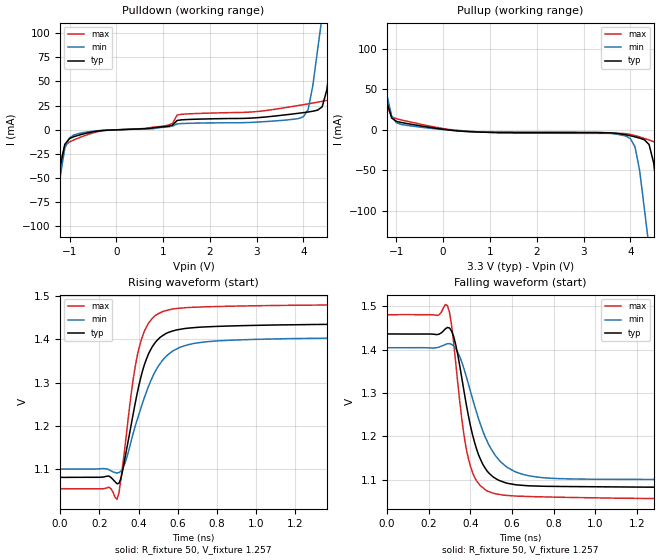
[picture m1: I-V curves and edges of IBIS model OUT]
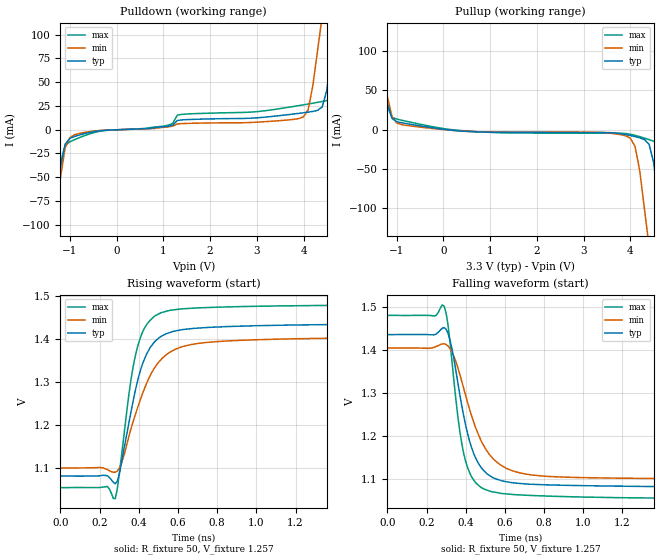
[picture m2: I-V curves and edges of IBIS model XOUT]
[IBIS Ver]   3.2
[Comment Char]   |_char
[File name]   vg3225vfn_lvds.ibs
[File Rev]   1.0
[Date]   2019/07/25 5:37:50
[Source]
[Notes]
[Disclaimer]
Seiko Epson Corporation makes no warranty with respect to the information
contained herein.
[Copyright]
Copyright(C) 2016, Seiko Epson Corporation. All rights reserved.
[Component]   vg3225vfn
Si_location Pin
Timing_location Pin
[Manufacturer]   Seiko Epson Corporation
[Package]
R_pkg   0.048   NA   NA
L_pkg   0.48n   NA   NA
C_pkg   0.21p   NA   NA
[Pin] signal_name   model_name   R_pin   L_pin   C_pin
1   VC   NC
2   OE   NC
3   GND   GND
4   OUT   OUT   0.048   0.48n   0.21p
5   XOUT   XOUT   0.048   0.48n   0.21p
6   VCC   POWER
[Diff Pin] inv_pin vdiff   tdelay_typ
4   5   0   0
| Models and submodels in the file (2): OUT (Output), XOUT (Output)
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[Model]   OUT
Model_type Output
Enable Active-High
Polarity Non-Inverting
Vref=1.250
Vmeas=1.250
Rref=50
Cref=0
C_comp   2.5p   2.5p   2.5p
[Temperature Range] 25   105   -40
[Voltage Range]   3.3   3.0   3.6
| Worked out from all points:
|   slope of the pulldown table from 0 to 0.495 V, typ, clamps not added: 525 ohm
|   slope of the pullup table from 0 to 0.495 V, typ, clamps not added: 178 ohm
|   falling waveform, R_fixture 50, V_fixture 1.257: 20-80 % time 95.8ps typ, 136ps min, 71.1ps max; typ from 1.44 V to 1.08 V
|   rising waveform, R_fixture 50, V_fixture 1.257: 20-80 % time 108ps typ, 149ps min, 84.3ps max; typ from 1.08 V to 1.44 V
[Pullup]
-3.3V     902.7mA    802.4mA    1.011A
-1.5V     156.5mA    150.6mA    165.7mA
-1.4V     115.1mA    114.4mA    118.8mA
-1.2V     33.42mA    42.1mA     29.33mA
-1V       10.35mA    8.744mA    13.55mA
3.9V      -6.214mA   -7.781mA   -4.855mA
4.1V      -8.8mA     -21.11mA   -7.16mA
4.3V      -12.42mA   -97.71mA   -10.64mA
4.5V      -41.27mA   -192.6mA   -14.74mA
4.7V      -144.8mA   -287.5mA   -20.73mA
5V        -306.1mA   -429.9mA   -148.7mA
6.6V      -1.166A    -1.189A    -1.111A
[Pulldown]
-3.3V     -1.17A     -1.051A    -1.295A
-1.4V     -142.7mA   -143.7mA   -146.1mA
-1.3V     -88.9mA    -96.14mA   -85.92mA
-1.2V     -38.72mA   -49.22mA   -34.15mA
-1.1V     -15.04mA   -18.91mA   -16.41mA
-900mV    -7.065mA   -5.272mA   -10.42mA
3.9V      17.07mA    11.65mA    25.14mA
4.1V      18.37mA    21.03mA    26.78mA
4.4V      23.74mA    118.1mA    29.41mA
4.7V      122.4mA    226.4mA    33.54mA
5V        246.7mA    334.8mA    131.6mA
6.6V      911.6mA    915mA      886.2mA
[Falling Waveform]
R_fixture=50
V_fixture=1.257
V_fixture_min=1.251
V_fixture_max=1.265
0s        1.436V     1.405V     1.481V
290ps     1.452V     1.414V     1.502V
330ps     1.411V     1.402V     1.368V
360ps     1.331V     1.37V      1.236V
390ps     1.249V     1.322V     1.149V
430ps     1.17V      1.255V     1.097V
480ps     1.12V      1.189V     1.074V
580ps     1.091V     1.127V     1.063V
740ps     1.085V     1.105V     1.06V
2ns       1.081V     1.1V       1.054V
[Rising Waveform]
R_fixture=50
V_fixture=1.257
V_fixture_min=1.251
V_fixture_max=1.265
0s        1.08V      1.099V     1.054V
250ps     1.083V     1.098V     1.058V
290ps     1.066V     1.091V     1.029V
310ps     1.078V     1.095V     1.078V
370ps     1.221V     1.178V     1.3V
400ps     1.29V      1.224V     1.376V
450ps     1.366V     1.291V     1.437V
520ps     1.408V     1.35V      1.464V
760ps     1.429V     1.395V     1.476V
2ns       1.436V     1.404V     1.481V
[Ramp]
R_load=50
dV/dt_r   2.136E-1/1.081E-10   1.826E-1/1.489E-10   2.563E-1/8.449E-11
dV/dt_f   2.136E-1/9.611E-11   1.826E-1/1.354E-10   2.563E-1/7.136E-11
|[End   OUT
[Model]   XOUT
Model_type Output
Enable Active-High
Polarity Inverting
Vref=1.250
Vmeas=1.250
Rref=50
Cref=0
C_comp   2.5p   2.5p   2.5p
[Temperature Range] 25   105   -40
[Voltage Range]   3.3   3.0   3.6
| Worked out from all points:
|   slope of the pulldown table from 0 to 0.495 V, typ, clamps not added: 525 ohm
|   slope of the pullup table from 0 to 0.495 V, typ, clamps not added: 178 ohm
|   falling waveform, R_fixture 50, V_fixture 1.257: 20-80 % time 103ps typ, 145ps min, 75.5ps max; typ from 1.44 V to 1.08 V
|   rising waveform, R_fixture 50, V_fixture 1.257: 20-80 % time 111ps typ, 154ps min, 87.1ps max; typ from 1.08 V to 1.44 V
[Pullup]
-3.3V     914.5mA    811.5mA    1.026A
-1.5V     158.5mA    152.3mA    168.2mA
-1.4V     116.6mA    115.7mA    120.5mA
-1.2V     33.75mA    42.57mA    29.56mA
-1V       10.34mA    8.742mA    13.52mA
3.9V      -6.216mA   -7.786mA   -4.856mA
4.1V      -8.805mA   -21.3mA    -7.164mA
4.3V      -12.44mA   -100.3mA   -10.65mA
4.5V      -42.16mA   -197.7mA   -14.76mA
4.7V      -149.2mA   -295.1mA   -20.79mA
5V        -315.5mA   -441.4mA   -153.9mA
6.6V      -1.202A    -1.221A    -1.151A
[Pulldown]
-3.3V     -1.206A    -1.079A    -1.341A
-1.4V     -147.1mA   -147.6mA   -151.4mA
-1.3V     -91.7mA    -98.73mA   -89.07mA
-1.2V     -39.66mA   -50.47mA   -34.94mA
-1.1V     -15.19mA   -19.12mA   -16.6mA
-900mV    -7.115mA   -5.297mA   -10.53mA
3.9V      17.18mA    11.69mA    25.38mA
4.1V      18.48mA    21.16mA    27.02mA
4.4V      23.9mA     119.4mA    29.67mA
4.7V      124.1mA    229mA      33.82mA
5V        250mA      338.6mA    133.8mA
6.6V      923.8mA    925.6mA    899.7mA
[Falling Waveform]
R_fixture=50
V_fixture=1.257
V_fixture_min=1.251
V_fixture_max=1.265
0s        1.436V     1.404V     1.48V
290ps     1.452V     1.414V     1.502V
330ps     1.403V     1.395V     1.373V
360ps     1.324V     1.358V     1.245V
390ps     1.246V     1.31V      1.159V
430ps     1.173V     1.247V     1.104V
490ps     1.12V      1.179V     1.077V
580ps     1.096V     1.132V     1.066V
740ps     1.087V     1.109V     1.061V
2ns       1.08V      1.099V     1.054V
[Rising Waveform]
R_fixture=50
V_fixture=1.257
V_fixture_min=1.251
V_fixture_max=1.265
0s        1.08V      1.099V     1.053V
240ps     1.081V     1.095V     1.056V
280ps     1.062V     1.089V     1.027V
300ps     1.084V     1.098V     1.085V
360ps     1.23V      1.191V     1.305V
390ps     1.296V     1.235V     1.376V
440ps     1.365V     1.297V     1.434V
510ps     1.405V     1.351V     1.461V
800ps     1.428V     1.394V     1.475V
2ns       1.435V     1.404V     1.48V
[Ramp]
R_load=50
dV/dt_r   2.131E-1/1.116E-10   1.822E-1/1.533E-10   2.563E-1/8.736E-11
dV/dt_f   2.131E-1/1.025E-10   1.822E-1/1.445E-10   2.563E-1/7.570E-11
|[End   XOUT
